| GHH_DESIGN_SPEC   IBIS MODEL
[IBIS Ver]   3.2
[File Name]   sprm153a.ibs
[File Rev]   1.01
[Date]   Mar 23, 2004
[Source]   Data created at ZUKEN
[Notes]   File originated from TISPICE Simulation.
|   Feb 3, 2003 : First release
|   Mar 23,2004 : Second release (rev 1.01) - $MH$
|   Notes:
|   -Some IV curves contain Non monotonic data points. They are
|   appropriate calculation results.
|   -Extreme current warnings are not the problem. The currents
|   correspond to the results of SPICE simulation.
|   -The warnings of 'value never becomes zero' are due to
|   IV curves which do not pass the zero voltage level. They are
|   not the problem, are caused by a voltage shift due to an
|   active resistor function.
|   -Some input cells do not have a power clamp diode. In this
|   case, current level in [POWER_Clamp] table is very low.
|   -This model contains a submodel definition. If your simulator
|   stops due to the errors, please follow instructions which
|   the simulator indicated, or remove the submodel section.
|   -Rev1.0 used internal package pins.  Corrected by replacing
|   internal package pin ID with BGA ball#
[Disclaimer]   Please be aware that in the absence of a written agreement
|   Texas Instruments(TI) assumes no liability for:
|   (1) The accuracy of the IBIS models provided to your company
|   (2) The proper functioning of these Models in your design
|   or for any resulting applications;or property rights
|   resulting from your use of these models. TI provides IBIS
|   Models as a service to our customers and therefore reserves
|   the right to limit distribution of the Models.
[Copyright]   Property of Texas Instruments Incorporated.
|   Unauthorised reproduction and/or distribution is strictly
|   prohibited. This product is protected under copyright law and
|   trade secret law as an unpublished work.
|   Created 1999,(C) Copyright 1999-2001,
|   Texas Instruments Incorporated., All Rights Reserved.
| Component   C5509_GHH
[Component]   C5509_GHH
[Manufacturer]   Texas Instruments
[Package]
| variable   typ   min   max
R_pkg   1.401820e-001  5.562165e-002  2.454900e-001
L_pkg   4.199604e-009  2.406723e-009  7.721048e-009
C_pkg   2.198809e-013  9.032977e-014  3.477553e-013
[Pin]  signal_name  model_name   R_pin   L_pin   C_pin
B2   VDD   POWER   1.5936E-01   4.3433E-09   2.0801E-13
B1   VSS   GND   1.4171E-01   3.7877E-09   1.6001E-13
C2   VSS   GND   1.2924E-01   3.6171E-09   2.1577E-13
C1   pu   OUI831   1.2593E-01   3.3377E-09   1.4759E-13
D4   dp   UIS245_UIS246_UOS181  1.6549E-01   5.0524E-09   2.6263E-13
D3   dn   UIS245_UIS246_UOS181  1.5017E-01   4.4020E-09   2.3552E-13
D2   VDDSHV2   POWER   1.2246E-01   3.4418E-09   2.0470E-13
D1   gpio7   IDG091_OUI831   1.2030E-01   3.2207E-09   1.6108E-13
E4   VSS   GND   1.0873E-01   4.5460E-09   2.6729E-13
E3   VDDSHV   POWER   8.7462E-02   3.7036E-09   2.3326E-13
E2   gpio2   IDG091_OUI831   1.1504E-01   3.2484E-09   1.9888E-13
E1   gpio1   IDG091_OUI831   1.1249E-01   3.0346E-09   1.5649E-13
F4   VSS   GND   1.0426E-01   4.3547E-09   2.6100E-13
F3   gpio0   IDG091_OUI831   1.3264E-01   3.9551E-09   2.1720E-13
|F2   x2clkin   UIS471   1.0832E-01   3.1000E-09   1.9384E-13
|F1   x1   UOS339   1.0649E-01   2.8737E-09   1.5230E-13
F5   clkout   OUKB31   1.6567E-01   5.3054E-09   2.7593E-13
G5   c0   OUI831_UPS239ON   1.6591E-01   5.3265E-09   2.7149E-13
G2   c1   OUI831   1.0294E-01   2.9503E-09   1.7619E-13
G1   VDD   POWER   5.5622E-02   2.4067E-09   1.5492E-13
G3   a20   OUI831   1.2531E-01   3.7725E-09   2.2006E-13
G4   c2   OUI831_UPS239ON   1.4489E-01   4.5225E-09   2.4319E-13
H3   a19   OUI831   1.2511E-01   3.7681E-09   2.1973E-13
H1   c3   IDG091_OUI831   1.0272E-01   2.7893E-09   1.4905E-13
H2   VDDSHV   POWER   1.0299E-01   2.9547E-09   1.7775E-13
H4   c4   OUI831_UPS239ON   1.4692E-01   4.5451E-09   2.3807E-13
H5   c5   OUI831_UPS239ON   1.6562E-01   5.3170E-09   2.7651E-13
J1   c6   OUI831_UPS239ON   1.0497E-01   2.8358E-09   1.5112E-13
J2   VDDSHV   POWER   5.7540E-02   2.6078E-09   1.8582E-13
J3   c7   OUI831_UPS239ON   1.3045E-01   3.8643E-09   2.1776E-13
J4   c8   OUI831_UPS239ON   1.5099E-01   4.6809E-09   2.5240E-13
K1   a18   OUI831   1.1020E-01   2.9773E-09   1.5501E-13
K2   c9   OUI831_UPS239ON   1.1228E-01   3.1800E-09   1.9715E-13
K3   c11   OUI831_UPS239ON   1.3808E-01   4.0893E-09   2.2611E-13
J5   VDD   POWER   1.9610E-01   6.3156E-09   3.1011E-13
L1   VDD   POWER   1.2154E-01   3.3081E-09   1.7721E-13
L2   c14   OUI831_UPS239ON   1.2403E-01   3.5078E-09   2.0687E-13
L3   c12   OUI831_UPS239ON   1.4909E-01   4.3768E-09   2.3396E-13
K4   VSS   GND   1.2803E-01   5.3096E-09   2.9498E-13
M1   c10   OUI831_UPS239ON   1.2873E-01   3.4180E-09   1.4897E-13
M2   c13   OUI831_UPS239ON   1.3202E-01   3.6866E-09   2.1705E-13
K5   VSS   GND   2.2786E-01   7.2951E-09   3.3542E-13
N1   VSS   GND   1.4172E-01   3.7921E-09   1.6041E-13
P1   VSS   GND   1.6685E-01   4.6413E-09   2.0950E-13
N2   VSS   GND   1.6725E-01   4.5610E-09   2.1197E-13
P2   VSS   GND   1.5636E-01   4.1509E-09   1.8354E-13
M3   VSS   GND   1.7596E-01   5.0469E-09   2.5091E-13
N3   a13   OUI831_UPS239ON   1.4835E-01   4.0944E-09   2.2804E-13
P3   a12   OUI831_UPS239ON   1.4652E-01   3.8558E-09   1.7412E-13
L4   a11   OUI831_UPS239ON   1.8712E-01   5.6173E-09   2.7879E-13
M4   VDD   POWER   1.0263E-01   4.3120E-09   2.5583E-13
N4   a10   OUI831_UPS239ON   1.4213E-01   3.9406E-09   2.1900E-13
P4   a9   OUI831_UPS239ON   1.4073E-01   3.7359E-09   1.7582E-13
L5   a8   OUI831_UPS239ON   1.8169E-01   5.4770E-09   2.7486E-13
M5   VSS   GND   9.7693E-02   4.1148E-09   2.4790E-13
N5   a7   OUI831_UPS239ON   1.3514E-01   3.7584E-09   2.1268E-13
P5   a17   OUI831   1.3320E-01   3.5575E-09   1.7147E-13
L6   a6   OUI831_UPS239ON   1.7438E-01   5.2704E-09   2.6899E-13
M6   a5   OUI831_UPS239ON   1.5273E-01   4.4603E-09   2.3147E-13
N6   VDDSHV   POWER   7.0623E-02   3.1291E-09   2.1482E-13
P6   a4   OUI831_UPS239ON   1.3165E-01   3.4614E-09   1.7628E-13
K6   a3   OUI831_UPS239ON   1.8842E-01   5.8761E-09   2.9210E-13
K7   a2   OUI831_UPS239ON   1.8895E-01   5.9014E-09   2.8807E-13
N7   VDD   POWER   6.8987E-02   3.0641E-09   2.0039E-13
P7   a16   OUI831   1.2672E-01   3.3897E-09   1.6619E-13
M7   a1   OUI831_UPS239ON   1.4913E-01   4.3672E-09   2.3704E-13
L7   a0   OUI831_UPS239ON   1.6887E-01   5.1216E-09   2.6016E-13
M8   a15   OUI831_UPS239ON   1.4918E-01   4.3701E-09   2.3683E-13
P8   VDDSHV   POWER   6.7729E-02   2.8847E-09   1.7294E-13
N8   VDD   POWER   1.2618E-01   3.5166E-09   1.9413E-13
L8   d0   OUI831_UPS239ON   1.7061E-01   5.1439E-09   2.5593E-13
K8   d1   OUI831_UPS239ON   1.9005E-01   5.9318E-09   2.9413E-13
P9   d2   OUI831_UPS239ON   1.2928E-01   3.4463E-09   1.6867E-13
N9   VSS   GND   7.0380E-02   3.1238E-09   2.0412E-13
M9   d3   OUI831_UPS239ON   1.5486E-01   4.4801E-09   2.3526E-13
L9   d4   OUI831_UPS239ON   1.7523E-01   5.2916E-09   2.6958E-13
P10   d5   OUI831_UPS239ON   1.3403E-01   3.5741E-09   1.7176E-13
N10   VSS   GND   7.3350E-02   3.2240E-09   2.1877E-13
M10   d6   OUI831_UPS239ON   1.5991E-01   4.6401E-09   2.4095E-13
K9   a14   OUI831_UPS239ON   2.1687E-01   6.8409E-09   3.2470E-13
P11   d7   OUI831_UPS239ON   1.4126E-01   3.8058E-09   1.9168E-13
N11   d8   OUI831_UPS239ON   1.4271E-01   3.9543E-09   2.1936E-13
M11   VDD   POWER   1.0146E-01   4.2634E-09   2.5274E-13
L10   d9   OUI831_UPS239ON   2.0425E-01   6.2768E-09   3.0306E-13
P12   d10   OUI831_UPS239ON   1.4762E-01   3.8895E-09   1.6309E-13
N12   d11   OUI831_UPS239ON   1.5040E-01   4.1461E-09   2.2885E-13
K10   VDDSHV   POWER   2.4549E-01   7.7210E-09   3.4776E-13
P13   VDDSHV   POWER   1.5871E-01   4.2088E-09   1.7299E-13
P14   VDDSHV   POWER   1.7852E-01   4.9442E-09   2.0863E-13
N13   VDDSHV   POWER   1.6151E-01   4.3949E-09   2.0964E-13
N14   VSS   GND   1.4170E-01   3.7838E-09   1.7325E-13
M12   VDDSHV   POWER   1.6032E-01   4.6300E-09   2.3861E-13
M13   VSS   GND   1.3198E-01   3.6855E-09   2.1741E-13
M14   d12   OUI831_UPS239ON   1.2875E-01   3.4160E-09   1.4970E-13
L11   d13   OUI831_UPS239ON   1.6821E-01   5.1251E-09   2.6422E-13
L12   d14   OUI831_UPS239ON   1.4662E-01   4.3081E-09   2.3314E-13
L13   d15   OUI831_UPS239ON   1.2160E-01   3.4200E-09   2.0380E-13
L14   VDD   POWER   6.5470E-02   2.7742E-09   1.6892E-13
K11   emu0   IDG041OUI831PS1001ON  1.6184E-01   4.9748E-09   2.6086E-13
K12   emu1   IDG041OUI831PS1001ON  1.3827E-01   4.0939E-09   2.2595E-13
K13   tdo   OUI831   1.1246E-01   3.1844E-09   1.9677E-13
K14   tdi   IDG041_PS1001ON   1.1034E-01   2.9825E-09   1.5531E-13
J11   VDD   POWER   1.0317E-01   4.3122E-09   2.5951E-13
J12   trstn   IDG041_PE1001ON   1.3067E-01   3.9063E-09   2.1576E-13
J13   tck   IDG091_PS1001ON   1.0636E-01   3.0373E-09   1.9220E-13
J14   tms   IDG041_PS1001ON   1.0515E-01   2.8409E-09   1.5123E-13
J10   VDD   POWER   1.1891E-01   4.9134E-09   2.8047E-13
H10   VDDSHV   POWER   1.1967E-01   4.9502E-09   2.7730E-13
H13   sda   IDI091_UOS205   1.0439E-01   2.9975E-09   1.7792E-13
H14   scl   IDI091_UOS205   1.0370E-01   2.8099E-09   1.4928E-13
H12   nreset   IDG091   1.2575E-01   3.7845E-09   2.2020E-13
H11   a0e   OUI831   1.4508E-01   4.5282E-09   2.4333E-13
G12   VSS1   GND   1.2557E-01   3.7791E-09   2.1998E-13
G14   nint0   IDG091   1.0264E-01   2.7877E-09   1.4929E-13
G13   nint1   IDG091   1.0180E-01   2.9069E-09   1.7690E-13
G11   VDD1   POWER   1.4560E-01   4.5206E-09   2.3799E-13
G10   nint2   IDG091   1.6477E-01   5.2946E-09   2.7586E-13
F14   nint3   IDG091   1.0359E-01   2.8022E-09   1.4986E-13
F13   VDDSHV   POWER   1.0357E-01   2.9696E-09   1.8063E-13
F12   nint4   IDG091   1.2796E-01   3.8120E-09   2.1648E-13
F11   VSS   GND   1.4852E-01   4.6194E-09   2.5053E-13
E14   xf   OUI831   1.0726E-01   2.8972E-09   1.5338E-13
E13   VSS   GND   1.0928E-01   3.1099E-09   1.9501E-13
E12   VSS3V   GND   8.3406E-02   3.5517E-09   2.2819E-13
F10   VDD3VHV   POWER   1.9019E-01   6.1674E-09   3.0579E-13
|D14   ain0   SW0101   1.1520E-01   3.1482E-09   1.7298E-13
|D13   ain1   SW0101   1.1729E-01   3.3394E-09   2.0277E-13
|D12   ain2   SW0101   1.4440E-01   4.2595E-09   2.3062E-13
|C14   ain3   SW0101   1.8218E-01   5.7199E-09   2.8714E-13
C13   VDDAHV   POWER   1.2621E-01   3.3545E-09   1.4744E-13
B14   VSSA   GND   1.2938E-01   3.6207E-09   2.1553E-13
A14   VDD5   POWER   1.7345E-01   4.7483E-09   2.1828E-13
B13   VDD5   POWER   1.6990E-01   4.6277E-09   2.1387E-13
A13   VDD5   POWER   1.5950E-01   4.2346E-09   1.7308E-13
C12   VDD4   POWER   1.7954E-01   5.1369E-09   2.5301E-13
|B12   rtcx2   OS11V1   1.5378E-01   4.2316E-09   2.3164E-13
|A12   rtcx1   OS11H1   1.5337E-01   4.0283E-09   1.8641E-13
D11   VSS   GND   1.9621E-01   5.8456E-09   2.8480E-13
C11   VSS   GND   1.7483E-01   5.0199E-09   2.5342E-13
B11   VSS   GND   1.4780E-01   4.0817E-09   2.2306E-13
A11   s23   OUI831_UPS239ON   1.4601E-01   3.8685E-09   1.7985E-13
D10   s25   IDG041_OUI831   1.8655E-01   5.5982E-09   2.7862E-13
C10   VDD   POWER   1.0044E-01   4.2245E-09   2.5128E-13
B10   s24   IDG091_OUI831   1.4011E-01   3.8812E-09   2.1676E-13
A10   s21   IDG041_OUI831   1.3821E-01   3.6838E-09   1.7433E-13
D9   VDDSHV1   POWER   1.7885E-01   5.3803E-09   2.7165E-13
C9   s22   IDG041_OUI831   1.5698E-01   4.5658E-09   2.3450E-13
B9   VSS   GND   1.3314E-01   3.7259E-09   2.1114E-13
A9   s20   IDG091_OUI831   1.3128E-01   3.4992E-09   1.6995E-13
E9   s13   OUI831_UPS239ON   1.9045E-01   5.9275E-09   2.9356E-13
E8   s15   IDG041_OUI831   1.9066E-01   5.9502E-09   2.8937E-13
B8   VDD   POWER   1.2787E-01   3.7259E-09   9.0330E-14
A8   VDDSHV1   POWER   1.2739E-01   3.4040E-09   1.6679E-13
C8   s14   IDG091_OUI831   1.4932E-01   4.3728E-09   2.3718E-13
D8   s11   IDG041_OUI831   1.6894E-01   5.1240E-09   2.6018E-13
C7   VSS   GND   1.4915E-01   4.3692E-09   2.3681E-13
A7   s12   IDG041_OUI831   1.2672E-01   3.3898E-09   1.6593E-13
B7   VDD   POWER   1.2615E-01   3.5159E-09   1.9405E-13
D7   s10   IDG091_OUI831   1.7036E-01   5.1389E-09   2.5578E-13
E7   dx0   OUI831   1.8979E-01   5.9257E-09   2.9380E-13
A6   VDD   POWER   6.8539E-02   2.9178E-09   1.7458E-13
B6   fsx0   IDG041_OUI831   1.2800E-01   3.5844E-09   1.9827E-13
C6   clkx0   IDG091_OUI831   1.5322E-01   4.4428E-09   2.3434E-13
D6   dr0   IDG041   1.7359E-01   5.2494E-09   2.6839E-13
A5   fsr0   IDG041_OUI831   1.3213E-01   3.5230E-09   1.7108E-13
B5   clkr0   IDG091_OUI831   1.3385E-01   3.7285E-09   2.1228E-13
C5   VSS   GND   9.6524E-02   4.0783E-09   2.4658E-13
E6   VDDSHV1   POWER   2.1498E-01   6.7942E-09   3.2302E-13
A4   VDDSHV1   POWER   1.3968E-01   3.7667E-09   1.9015E-13
B4   tinout0   IDG091_OUI831   1.3748E-01   3.8253E-09   2.1480E-13
C4   gpio6   IDG091_OUI831   1.6442E-01   4.7665E-09   2.4203E-13
D5   gpio5   OUI831_UPS239ON   1.9972E-01   6.1411E-09   2.9866E-13
A3   gpio4   IDG091_OUI831   1.4467E-01   3.8103E-09   1.9540E-13
B3   gpio3   IDG091_OUI831   1.4742E-01   4.0716E-09   2.2656E-13
E5   VSS   GND   2.4140E-01   7.5951E-09   3.4626E-13
A2   VSS   GND   1.6737E-01   4.5201E-09   1.9075E-13
[Diff Pin] inv_pin   vdiff   tdelay_typ   tdelay_min   tdelay_max
D4   D3   0.2   NA   NA   NA
| Models and submodels in the file (14): OUI831 (3-state), OUKB31 (3-state), IDG091 (Input), IDG041 (Input), IDG041_PS1001ON (Input), IDG091_PS1001ON (Input), IDG041_PE1001ON (Input), IDI091_UOS205 (I/O_open_drain), IDG041OUI831PS1001ON (I/O), IDG091_OUI831 (I/O), OUI831_UPS239ON (I/O), UPS239BH (Bus_hold), IDG041_OUI831 (I/O), UIS245_UIS246_UOS181 (I/O)
